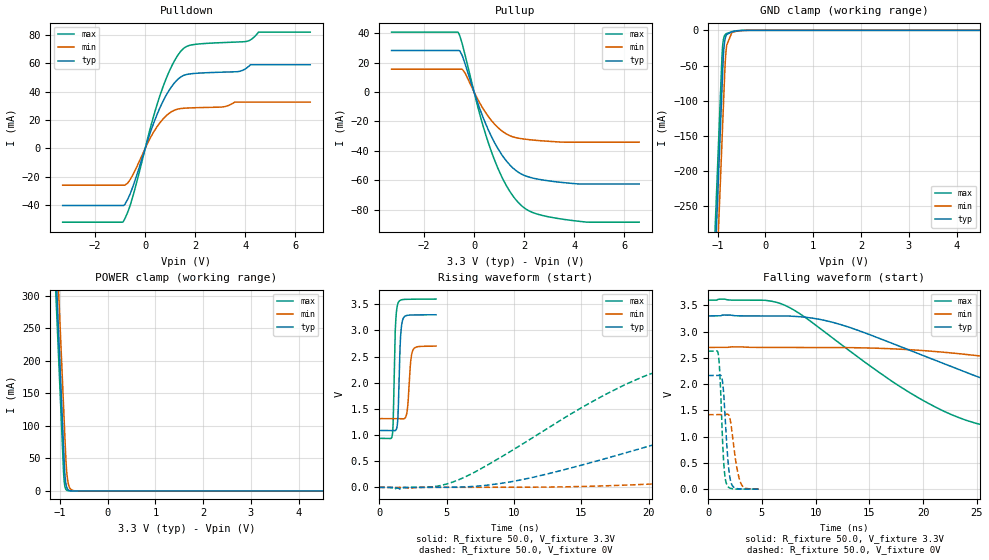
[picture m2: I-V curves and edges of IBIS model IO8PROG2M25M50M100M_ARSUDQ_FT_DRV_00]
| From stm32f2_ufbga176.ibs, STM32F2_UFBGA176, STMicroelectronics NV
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| *** New cell (Generated with 5.14beta1 (Sep 20 2010 13:23:23))
[Model]   IO8PROG2M25M50M100M_ARSUDQ_FT_DRV_00
Model_type 3-state
Polarity   Non-Inverting
Enable   Active-Low
| CAP_THRESHOLD on pad IOV33 is "CMOS" :
| Rising=10.0% of vddio   Falling=90.0% of vddio
| C_comp min and max val. don't necessarily correlate with the min and max pvt
| but are the smallest and greatest pad capacitance found.
| var   typ   min   max
C_comp   2.14325pF  2.03775pF  2.26775pF
Vmeas = 1.65V   | Reference voltage for timing measurements
Cref  = 50.0pF   | Timing specification test load capacitance value
Rref  = 10.0MOhm   | Timing specification test load resistance value
Vref  = 1.65V   | Timing specification test load voltage
[Model Spec]
| variable   typ   min   max
[Temperature Range] 25.0 125.0 -40.0
| variable   typ   min   max
[Voltage Range] 3.3V 2.7V 3.6V
| variable   typ   min   max
[POWER Clamp Reference] 3.3V 2.7V 3.6V
| variable   typ   min   max
[GND Clamp Reference] 0V 0V 0V
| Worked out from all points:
|   slope of the pulldown table from 0 to 0.495 V, typ, clamps not added: 20 ohm
|   slope of the pullup table from 0 to 0.495 V, typ, clamps not added: 21.7 ohm
|   GND clamp passes 1 mA (typ) near -0.62 V on its own axis
|   POWER clamp passes 1 mA (typ) near -0.81 V on its own axis
|   rising waveform, R_fixture 50.0, V_fixture 3.3V: 20-80 % time 162ps typ, 212ps min, 145ps max; typ from 1.09 V to 3.3 V
|   falling waveform, R_fixture 50.0, V_fixture 3.3V: 20-80 % time 18.1ns typ, 35.4ns min, 11.7ns max; typ from 3.3 V to 1.09 V
|   rising waveform, R_fixture 50.0, V_fixture 0V: 20-80 % time 19.4ns typ, 44ns min, 10.8ns max; typ from 0 V to 2.17 V
|   falling waveform, R_fixture 50.0, V_fixture 0V: 20-80 % time 416ps typ, 600ps min, 329ps max; typ from 2.17 V to 0 V
[POWER Clamp]
-3.3V     4.11A      4.173A     4.072A
-1.09V    352.5mA    415.9mA    314.5mA
-1.05V    284.5mA    347.9mA    246.5mA
-1.01V    216.5mA    279.9mA    178.5mA
-920mV    63.51mA    126.9mA    25.85mA
-900mV    31.51mA    92.9mA     9.552mA
-890mV    21.35mA    75.9mA     5.807mA
-870mV    9.804mA    44.01mA    2.146mA
-840mV    3.05mA     18.36mA    482.1uA
-780mV    295.2uA    3.194mA    24.34uA
-660mV    2.764uA    96.54uA    62.42nA
6.6V      0A         0A         0A
[GND Clamp]
-3.3V     -4.149A    -4.223A    -4.103A
-1.06V    -340.6mA   -415.4mA   -294.5mA
-940mV    -136.6mA   -211.4mA   -90.54mA
-910mV    -85.55mA   -160.4mA   -39.54mA
-900mV    -68.55mA   -143.4mA   -26.55mA
-880mV    -36.73mA   -109.4mA   -13.46mA
-860mV    -19.54mA   -75.4mA    -8.234mA
-840mV    -11.29mA   -44.89mA   -5.954mA
-810mV    -6.008mA   -21.13mA   -4.401mA
-700mV    -1.958mA   -2.906mA   -1.882mA
-470mV    -105.5uA   -263.9uA   -47.31uA
6.6V      9.456nA    1.185uA    63.86pA
| variable   typ   min   max
[Pullup Reference] 3.3V 2.7V 3.6V
| variable   typ   min   max
[Pulldown Reference] 0V 0V 0V
[Pullup]
-3.3V     28.27mA    15.58mA    40.81mA
-630mV    28.27mA    15.58mA    40.39mA
-480mV    25.11mA    15.58mA    33.22mA
-350mV    18.69mA    12.64mA    24.51mA
240mV     -11.89mA   -7.822mA   -15.87mA
710mV     -30.8mA    -19.68mA   -41.36mA
1.3V      -47.02mA   -28.56mA   -63.9mA
1.65V     -53.05mA   -30.92mA   -72.82mA
2.01V     -56.71mA   -31.98mA   -78.86mA
2.7V      -59.67mA   -33.14mA   -83.8mA
3.9V      -62.11mA   -34.07mA   -87.29mA
6.6V      -62.54mA   -34.07mA   -88.51mA
[Pulldown]
-3.3V     -40.26mA   -25.94mA   -51.99mA
-870mV    -40.25mA   -25.94mA   -51.33mA
-700mV    -35.92mA   -24.51mA   -45.06mA
-470mV    -25.89mA   -17.87mA   -32.39mA
240mV     12.97mA    8.52mA     16.62mA
590mV     28.62mA    18.11mA    37.2mA
1.07V     43.85mA    26mA       58.31mA
1.54V     51.42mA    28.24mA    70.48mA
2.01V     52.82mA    28.63mA    73.27mA
4.01V     56.01mA    32.56mA    75.18mA
4.53V     58.89mA    32.56mA    81.88mA
6.6V      58.89mA    32.56mA    81.88mA
[Ramp]
dV/dt_r 1.29886V/19.41546ns 851.10443mV/44.02633ns 1.57728V/10.77909ns
dV/dt_f 1.3278V/18.12563ns 831.25489mV/35.44068ns 1.59819V/11.71704ns
R_load = 50.0
| Removed startup time: 0s 0s 0s  .
| Removed end time: 4.214ns.
[Rising Waveform]
R_fixture   = 50.0
V_fixture   = 3.3V
V_fixture_min = 2.7V
V_fixture_max = 3.6V
0s        1.087V     1.314V     936.3mV
980ps     1.087V     1.314V     1.006V
1.044ns   1.086V     1.314V     1.3V
1.204ns   1.086V     1.314V     3.057V
1.406ns   1.425V     1.314V     3.526V
1.576ns   2.826V     1.313V     3.577V
1.774ns   3.223V     1.308V     3.59V
2.08ns    3.287V     1.463V     3.594V
2.498ns   3.295V     2.619V     3.596V
4.218ns   3.299V     2.7V       3.599V
| Removed startup time: 0s 0s 0s  .
| Removed end time: 250.0ns.
[Falling Waveform]
R_fixture   = 50.0
V_fixture   = 3.3V
V_fixture_min = 2.7V
V_fixture_max = 3.6V
0s        3.3V       2.7V       3.6V
6.56ns    3.3V       2.7V       3.547V
11.52ns   3.181V     2.7V       2.889V
18ns      2.707V     2.665V     1.935V
23.08ns   2.298V     2.586V     1.382V
33.44ns   1.569V     2.328V     1.048V
46.92ns   1.236V     1.955V     974.1mV
62.96ns   1.147V     1.622V     949.4mV
84.64ns   1.108V     1.446V     940mV
250.1ns   1.087V     1.315V     936.3mV
| Removed startup time: 0s 0s 0s  .
| Removed end time: 247.48ns.
[Rising Waveform]
R_fixture   = 50.0
V_fixture   = 0V
V_fixture_min = 0V
V_fixture_max = 0V
0s        7.749nV    280.7nV    5.731nV
5.84ns    3.51mV     -128.9uV   138.7mV
11.36ns   188.3mV    2.766mV    944.3mV
20.72ns   841mV      69.51mV    2.222V
30.84ns   1.532V     241.1mV    2.543V
38.48ns   1.88V      402.7mV    2.595V
47.28ns   2.035V     600.8mV    2.616V
70.4ns    2.141V     1.047V     2.627V
95.52ns   2.16V      1.293V     2.629V
247.6ns   2.165V     1.419V     2.629V
| Removed startup time: 0s 0s 0s  .
| Removed end time: 4.762ns.
[Falling Waveform]
R_fixture   = 50.0
V_fixture   = 0V
V_fixture_min = 0V
V_fixture_max = 0V
0s        2.165V     1.419V     2.629V
960ps     2.166V     1.419V     2.557V
1.14ns    2.172V     1.419V     2.025V
1.36ns    2.021V     1.418V     871.2mV
1.526ns   1.592V     1.42V      320.7mV
1.722ns   901.9mV    1.426V     97.45mV
2.118ns   137.1mV    1.254V     14.39mV
2.612ns   14.53mV    485.2mV    3.191mV
3.03ns    4.284mV    120.4mV    1.97mV
4.766ns   437.3uV    300.5uV    606.9uV
